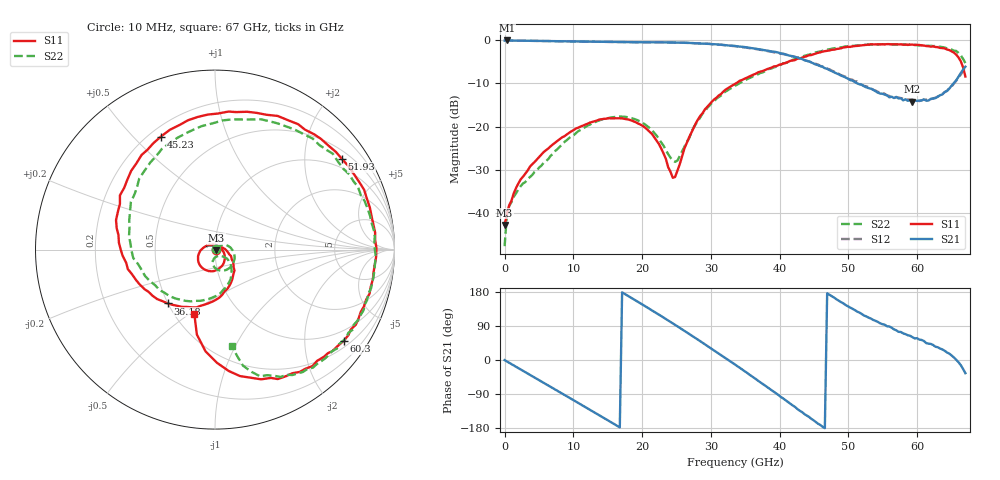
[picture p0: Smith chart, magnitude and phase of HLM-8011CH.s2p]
!Keysight Technologies,N5247B,US58420632,A.15.65.19
!Date: Tuesday, July 19, 2022 16:58:51
!Correction: S11(C  2-Port  )
!S21(C  2-Port  )
!S12(C  2-Port  )
!S22(C  2-Port  )
!S2P File: Measurements: S11, S21, S12, S22:
# Hz S  dB  R 50
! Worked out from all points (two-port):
!   201 points, 10 MHz to 67 GHz, reference 50 ohm
!   highest |S21| = -0.07 dB at 344.9 MHz (marker M1); lowest = -14.3 dB at 59.3 GHz (marker M2)
!   |S21| within 3 dB of the highest: start of sweep to 40.16 GHz
!   lowest |S11| = -42.8 dB at 10 MHz (marker M3), VSWR 1.01, Z = 50.7 - j0.331 ohm
!   |S11| at or under -10 dB: start of sweep to 33.65 GHz
!   |S22| runs from -47.7 to -0.9 dB; largest |S21 - S12| = 0.024
!   S11 on the Smith chart (normalised r, x): 10 MHz: 1.01, -0.01; 36.18 GHz: 0.50, -0.36; 45.23 GHz: 0.25, +0.60; 51.93 GHz: 0.72, +2.97; 60.3 GHz: 0.67, -3.01; 67 GHz: 0.62, -0.53
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1e7  -42.76 -26.7  -0.10 -0.3  -0.08 -0.1  -47.69 34.1
3.4495e8  -40.26 21.9  -0.07 -3.8  -0.08 -3.8  -40.36 20.0
2.35465e9  -32.21 19.0  -0.13 -25.2  -0.12 -25.2  -33.79 36.2
6.37405e9  -25.06 -23.6  -0.21 -67.5  -0.20 -67.5  -27.49 34.5
1.13983e10  -19.79 -71.8  -0.33 -120.6  -0.33 -120.6  -20.50 0.5
1.709245e10  -18.12 -125.7  -0.45 178.5  -0.45 178.6  -17.71 -55.4
2.245165e10  -24.06 168.1  -0.51 119.6  -0.52 119.4  -22.86 -101.2
2.47963e10  -31.68 65.7  -0.56 92.7  -0.58 92.7  -28.17 -70.0
2.74759e10  -20.34 -21.8  -0.67 61.2  -0.69 61.3  -20.25 -39.0
2.982055e10  -14.84 -56.8  -0.86 33.3  -0.85 33.1  -15.10 -59.5
3.3505e10  -10.13 -100.5  -1.33 -11.9  -1.39 -12.1  -10.55 -106.0
3.61846e10  -7.98 -131.3  -1.90 -45.9  -1.96 -46.1  -8.32 -144.1
4.053895e10  -5.40 175.8  -3.14 -101.8  -3.23 -101.4  -5.38 150.5
4.48933e10  -3.29 120.2  -5.38 -158.6  -5.28 -157.8  -3.06 91.2
4.522825e10  -3.12 115.5  -5.63 -163.3  -5.46 -162.7  -2.84 86.6
4.857775e10  -1.98 73.1  -7.92 156.5  -7.79 156.8  -1.68 48.6
5.192725e10  -1.22 35.5  -10.31 121.5  -10.37 120.9  -1.14 17.9
5.594665e10  -0.93 -2.6  -13.24 88.5  -12.93 85.6  -0.96 -12.2
5.929615e10  -1.02 -28.1  -14.25 60.2  -13.73 60.1  -1.15 -32.0
6.0301e10  -1.12 -35.3  -14.02 53.9  -14.09 51.7  -1.22 -37.4
6.465535e10  -2.30 -70.4  -11.23 16.8  -11.14 14.3  -1.95 -62.7
6.7e10  -8.42 -107.6  -6.15 -34.8  -6.41 -36.1  -5.30 -80.1
